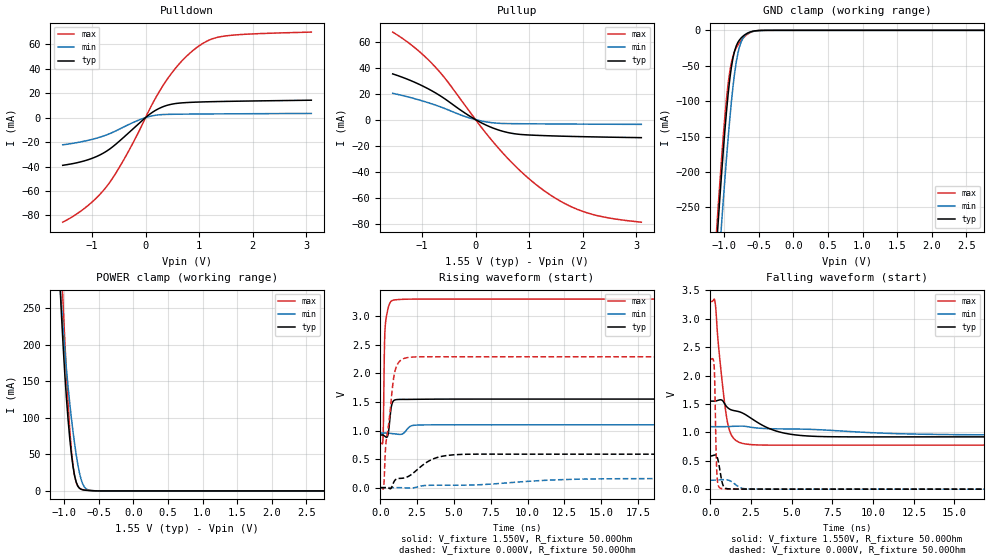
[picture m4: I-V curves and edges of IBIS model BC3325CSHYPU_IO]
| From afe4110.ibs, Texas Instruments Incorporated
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|   BC3325CSHYPU_IO model
[Model]   BC3325CSHYPU_IO
Model_type   I/O
Vinl = 0.465V  |0.275V for 1.1V
Vinh = 1.085V  |0.825V for 1.1V
Vmeas = 0.755V
Cref = 25pF   |15pF for 1.1V
|   typ   min   max
|   (NOM)   (WEAK)   (FAST)
C_comp   1.9304pF   1.785pF   1.9393pF
[Model Spec]
Vinl   0.465V   0.275V   0.99V
Vinh   1.085V   0.825V   2.31V
[Voltage Range]   1.550V   1.100V   3.300V
[Temperature Range]   27.0   85.0   0.0
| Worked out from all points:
|   slope of the pulldown table from 0 to 0.232 V, typ, clamps not added: 33.1 ohm
|   slope of the pullup table from 0 to 0.232 V, typ, clamps not added: 47.9 ohm
|   GND clamp passes 1 mA (typ) near -0.57 V on its own axis
|   POWER clamp passes 1 mA (typ) near -0.70 V on its own axis
|   falling waveform, V_fixture 1.550V, R_fixture 50.00Ohm: 20-80 % time 2.7ns typ, 7.68ns min, 568ps max; typ from 1.55 V to 0.92 V
|   rising waveform, V_fixture 1.550V, R_fixture 50.00Ohm: 20-80 % time 164ps typ, 321ps min, 106ps max; typ from 0.92 V to 1.55 V
|   rising waveform, V_fixture 0.000V, R_fixture 50.00Ohm: 20-80 % time 2.35ns typ, 8.23ns min, 550ps max; typ from 0 V to 0.586 V
|   falling waveform, V_fixture 0.000V, R_fixture 50.00Ohm: 20-80 % time 223ps typ, 475ps min, 102ps max; typ from 0.586 V to 0 V
[Pulldown]
|   Voltage   I(typ)   I(min)   I(max)
-1.55V    -38.99mA   -22.26mA   -85.48mA
-1.083V   -34.54mA   -18.64mA   -72.07mA
-708.8mV  -26.82mA   -13.79mA   -55.22mA
-334.9mV  -13.19mA   -6.094mA   -28.77mA
-31.16mV  -1.204mA   -453.4uA   -2.879mA
202.5mV   6.324mA    2.005mA    17.19mA
389.4mV   9.851mA    2.596mA    30.34mA
576.4mV   11.57mA    2.75mA     41.21mA
950.3mV   12.65mA    2.913mA    57.04mA
1.184V    12.95mA    2.984mA    63.24mA
1.464V    13.21mA    3.056mA    66.55mA
3.1V      14.21mA    3.402mA    69.88mA
[GND Clamp]
|   Voltage   I(typ)   I(min)   I(max)
-1.55V    -999.7mA   -1.05A     -993.8mA
-1.106V   -299.8mA   -370.2mA   -278.7mA
-1.083V   -266.2mA   -337mA     -244.6mA
-1.036V   -201.5mA   -272.3mA   -179.7mA
-989.2mV  -141.7mA   -210.4mA   -121.6mA
-942.5mV  -90.39mA   -152.7mA   -75.56mA
-872.4mV  -39.12mA   -79.9mA    -36.54mA
-825.6mV  -22.2mA    -45.43mA   -24.75mA
-778.9mV  -13.64mA   -23.63mA   -17.4mA
-685.4mV  -5.273mA   -6.116mA   -7.184mA
-428.4mV  -68.29uA   -124.7uA   -77.78uA
3.1V      0A         0A         0A
[Pullup]
|   Voltage   I(typ)   I(min)   I(max)
-1.55V    35.19mA    20.27mA    67.34mA
-1.129V   28.56mA    16mA       55.08mA
-755.5mV  20.71mA    11.27mA    40.59mA
-545.2mV  15.16mA    8.064mA    30.39mA
-124.6mV  3.107mA    1.452mA    6.934mA
272.6mV   -5.571mA   -2.156mA   -14.37mA
739.9mV   -10.91mA   -3.09mA    -35.57mA
1.207V    -12.16mA   -3.244mA   -52.36mA
1.651V    -12.74mA   -3.358mA   -64.13mA
2.072V    -13.14mA   -3.448mA   -71.47mA
2.563V    -13.51mA   -3.539mA   -76.08mA
3.1V      -13.84mA   -3.627mA   -78.85mA
[POWER Clamp]
|   Voltage   I(typ)   I(min)   I(max)
-1.55V    1.445A     1.342A     1.57A
-1.059V   281.2mA    282.7mA    353.1mA
-1.036V   236.7mA    250.1mA    301.4mA
-1.013V   195.7mA    220mA      251.5mA
-942.5mV  97.19mA    142.1mA    119.3mA
-895.7mV  51.02mA    100.1mA    56.39mA
-872.4mV  33.87mA    81.74mA    35.26mA
-825.6mV  12.13mA    49.62mA    11.47mA
-755.5mV  2.299mA    16.01mA    2.457mA
-685.4mV  860.2uA    3.089mA    1.144mA
-568.6mV  199.1uA    256.3uA    288.2uA
3.1V      0A         0A         -54.55pA
[Ramp]
R_load = 50.00Ohm
|   typ   min   max
dV/dt_r   351.379mV/2.352ns   94.846mV/8.219ns   1.374V/550.043ps
dV/dt_f   377.885mV/2.700ns   87.400mV/7.687ns   1.515V/567.610ps
[Falling Waveform]
V_fixture = 1.550V
V_fixture_min = 1.100V
V_fixture_max = 3.300V
R_fixture = 50.00Ohm
|   Time   V(typ)   V(min)   V(max)
0s        1.55V      1.1V       3.3V
300ps     1.55V      1.1V       3.279V
490ps     1.565V     1.1V       2.572V
770ps     1.554V     1.1V       1.785V
1.16ns    1.414V     1.103V     1.053V
1.59ns    1.375V     1.108V     853.3mV
2.52ns    1.246V     1.089V     783.8mV
4.61ns    982.6mV    1.06V      774.4mV
8.16ns    920.9mV    1.022V     774.6mV
125ns     920.2mV    954.3mV    774.6mV
[Rising Waveform]
V_fixture = 1.550V
V_fixture_min = 1.100V
V_fixture_max = 3.300V
R_fixture = 50.00Ohm
|   Time   V(typ)   V(min)   V(max)
0s        920.2mV    954.3mV    774.6mV
190ps     919.7mV    955.3mV    883.8mV
220ps     915.9mV    955.5mV    1.246V
290ps     903.8mV    955.9mV    2.537V
370ps     888.4mV    955.9mV    2.915V
540ps     945.6mV    953.6mV    3.146V
800ps     1.471V     946.4mV    3.273V
1.21ns    1.543V     934mV      3.291V
3.35ns    1.548V     1.099V     3.3V
125ns     1.55V      1.1V       3.3V
[Rising Waveform]
V_fixture = 0.000V
V_fixture_min = 0.000V
V_fixture_max = 0.000V
R_fixture = 50.00Ohm
|   Time   V(typ)   V(min)   V(max)
0s        56.99uV    71.9uV     22.07uV
230ps     871.5uV    14.26uV    -3.663mV
390ps     607uV      205.5uV    792.9mV
990ps     128.1mV    418.7uV    2.032V
1.36ns    162.6mV    153.9uV    2.223V
2.13ns    233.8mV    -6.928mV   2.284V
3.64ns    508.1mV    42.23mV    2.29V
5.98ns    584.8mV    44.94mV    2.29V
16.56ns   585.7mV    157.1mV    2.29V
125ns     585.7mV    158.1mV    2.29V
[Falling Waveform]
V_fixture = 0.000V
V_fixture_min = 0.000V
V_fixture_max = 0.000V
R_fixture = 50.00Ohm
|   Time   V(typ)   V(min)   V(max)
0s        585.7mV    158.1mV    2.29V
170ps     592.7mV    158.4mV    2.288V
240ps     598.4mV    159.3mV    2.158V
280ps     600.6mV    159.9mV    1.8V
370ps     591.6mV    161.1mV    547.1mV
440ps     550mV      162.1mV    149.2mV
550ps     402.6mV    163.6mV    32.29mV
810ps     53.68mV    167.5mV    7.265mV
3.17ns    639.5uV    967.8uV    56.69uV
125ns     56.99uV    71.9uV     22.07uV
